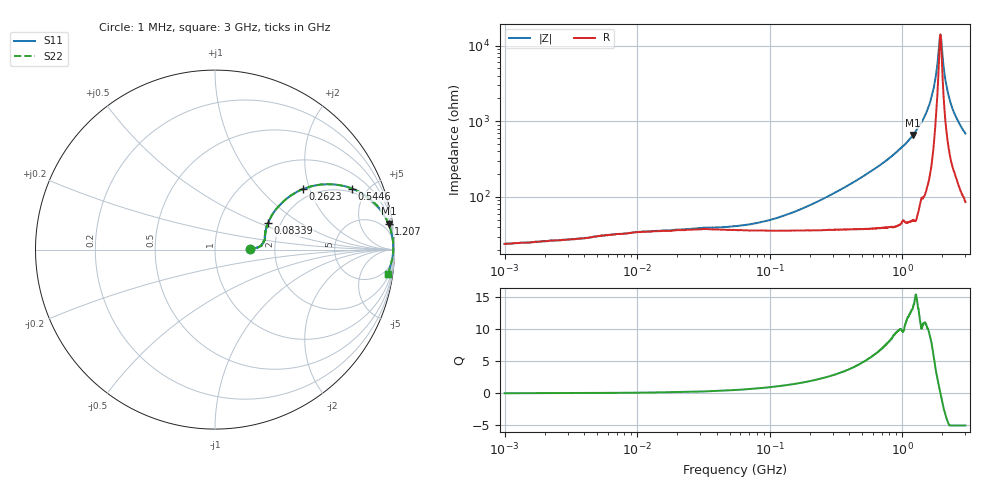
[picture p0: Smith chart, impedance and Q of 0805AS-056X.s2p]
!s-Parameter Generated by FASTRON Sdn. Bhd.
!FASTRON P/N : 0805AS-056X
!Keysight Technologies: E4991B_MY54100416_A.01.15
!Date: Mon Jun 15 12:51:12 2026
!Version  :Rev01  Mon Jun 15 12:51:12 2026
!Data & Calibration Information:
!Freq  S11  S21  S12  S22
!PortZ  Port1:50+j0  Port2:50+j0
!When reading reference impedance value at option line is always used.
! Remarks : This data is being provided solely for informational purposes.
# Hz S dB R 50
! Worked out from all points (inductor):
!   1601 points, 1 MHz to 3 GHz, reference 50 ohm
!   read as one part in series: L = 53.6 nH near 320.4 MHz
!   highest Q = 13.5 at 1.213 GHz (marker M1), where L = 86.6 nH
!   self-resonance near 1.941 GHz
!   S11 on the Smith chart (normalised r, x): 1 MHz: 1.48, +0.01; 83.39 MHz: 1.72, +0.57; 262.3 MHz: 1.73, +1.81; 544.6 MHz: 1.75, +3.97; 1.207 GHz: 2, +13; 3 GHz: 3, -14
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1000000  -14.30 0.7  -1.87 -0.2  -1.87 -0.2  -14.30 0.7
3804036  -13.10 2.1  -2.16 -0.6  -2.16 -0.6  -13.10 2.1
1.447069e7  -11.60 6.0  -2.65 -2.1  -2.65 -2.1  -11.60 6.0
5.504702e7  -10.50 19.5  -2.78 -7.9  -2.78 -7.9  -10.50 19.5
8.338914e7  -9.61 26.6  -2.86 -11.9  -2.86 -11.9  -9.61 26.6
2.083556e8  -5.67 35.5  -3.74 -27.7  -3.74 -27.7  -5.67 35.5
2.622844e8  -4.51 34.5  -4.28 -33.5  -4.28 -33.5  -4.51 34.5
5.445776e8  -1.55 24.0  -7.68 -55.3  -7.68 -55.3  -1.55 24.0
7.925923e8  -0.69 16.5  -10.80 -66.4  -10.80 -66.4  -0.69 16.5
1.206698e9  -0.20 8.6  -16.50 -77.2  -16.50 -77.2  -0.20 8.6
1.212752e9  -0.19 8.4  -16.60 -77.3  -16.60 -77.3  -0.19 8.4
1.45942e9  -0.10 5.1  -21.00 -79.7  -21.00 -79.7  -0.10 5.1
1.629261e9  -0.07 3.1  -25.20 -80.3  -25.20 -80.3  -0.07 3.1
1.75626e9  -0.06 1.8  -30.10 -76.5  -30.10 -76.5  -0.06 1.8
1.893158e9  -0.06 0.5  -39.50 -48.6  -39.50 -48.6  -0.06 0.5
1.941122e9  -0.06 0.0  -43.00 -4.9  -43.00 -4.9  -0.06 0.0
2.000286e9  -0.06 -0.5  -38.90 50.5  -38.90 50.5  -0.06 -0.5
2.092429e9  -0.07 -1.3  -32.30 70.0  -32.30 70.0  -0.07 -1.3
2.156205e9  -0.08 -1.9  -29.50 73.5  -29.50 73.5  -0.08 -1.9
2.301132e9  -0.10 -3.0  -25.40 76.2  -25.40 76.2  -0.10 -3.0
2.581816e9  -0.16 -5.1  -20.90 76.0  -20.90 76.0  -0.16 -5.1
3e9  -0.24 -8.1  -17.00 74.8  -17.00 74.8  -0.24 -8.1
